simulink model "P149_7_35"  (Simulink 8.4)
settings: Solver=ode45  StartTime=0.0  StopTime=10.0  RelTol=1e-3

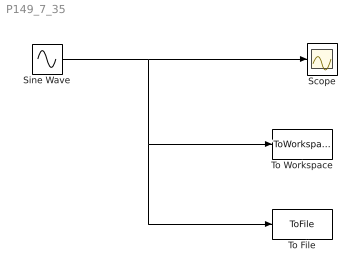
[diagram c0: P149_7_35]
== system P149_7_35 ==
  Scope : Scope
  Sine Wave : Sin  SampleTime=0
  To File : ToFile
  To Workspace : ToWorkspace  VariableName=simout  SampleTime=-1
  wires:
  Sine Wave/1 -> To File/1, To Workspace/1, Scope/1
